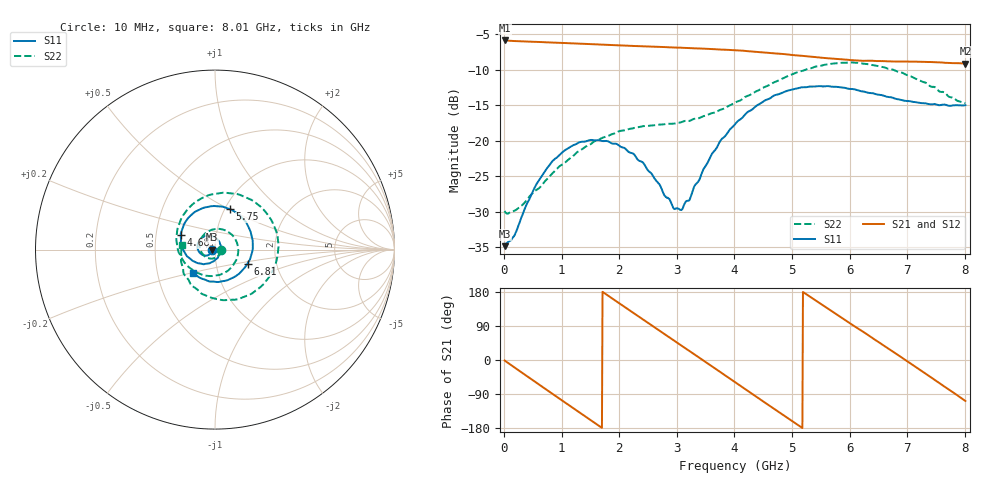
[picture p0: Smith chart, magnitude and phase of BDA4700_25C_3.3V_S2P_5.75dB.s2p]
!Agilent Technologies,E5071B,MY42404982,A.09.10
!Date: Mon Oct 20 18:05:24 2025
!Data & Calibration Information:
!Freq	S11:SOLT2(ON)	S21:SOLT2(ON)	S12:SOLT2(ON)	S22:SOLT2(ON)
# Hz S RI R 50
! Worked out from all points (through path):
!   801 points, 10 MHz to 8.01 GHz, reference 50 ohm
!   highest |S21| = -5.87 dB at 10 MHz (marker M1); lowest = -9.1 dB at 8.01 GHz (marker M2)
!   group delay of S21, straight-line fit = 286 ps
!   lowest |S11| = -34.8 dB at 10 MHz (marker M3), VSWR 1.04, Z = 48.2 - j0.106 ohm
!   |S11| at or under -10 dB: start of sweep to end of sweep
!   |S22| runs from -30.3 to -8.9 dB; largest |S21 - S12| = 0.0061
!   S11 on the Smith chart (normalised r, x): 10 MHz: 0.96, -0.00; 4.68 GHz: 0.67, +0.11; 5.75 GHz: 1.06, +0.51; 6.81 GHz: 1.42, -0.23; 8.01 GHz: 0.76, -0.20
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1e7  -0.0181 -0.0011  0.5086 -0.0111  0.5084 -0.0116  0.032 -0.00251
3.3e8  -0.0237 -0.02  0.4085 -0.2903  0.4083 -0.2903  0.023 -0.0273
7.1e8  -0.051 -0.0336  0.1238 -0.4786  0.1237 -0.4786  -0.0137 -0.0501
1.02e9  -0.0807 -0.0221  -0.1512 -0.4643  -0.1512 -0.4647  -0.0575 -0.0371
1.35e9  -0.0979 0.0111  -0.383 -0.2929  -0.383 -0.2934  -0.0853 0.0179
1.64e9  -0.0899 0.0467  -0.4732 -0.0599  -0.4733 -0.0597  -0.0673 0.0767
1.93e9  -0.0623 0.0724  -0.4339 0.1842  -0.4338 0.1845  -0.00695 0.1131
2.32e9  -0.0129 0.0727  -0.2082 0.4149  -0.208 0.415  0.0882 0.0881
2.68e9  0.0242 0.0441  0.0844 0.4508  0.0837 0.4506  0.1297 -0.00255
3.08e9  0.0304 -0.0118  0.3571 0.2776  0.3541 0.2797  0.0841 -0.1062
3.53e9  -0.0146 -0.0681  0.4391 -0.0656  0.4394 -0.0662  -0.0417 -0.1463
4.01e9  -0.111 -0.0694  0.2275 -0.3701  0.2281 -0.369  -0.1724 -0.0692
4.34e9  -0.1701 -0.0135  -0.0195 -0.4237  -0.0197 -0.4247  -0.2141 0.0439
4.68e9  -0.1913 0.0809  -0.2547 -0.3252  -0.254 -0.3266  -0.1848 0.1789
5.02e9  -0.1485 0.1769  -0.3838 -0.1169  -0.3851 -0.1174  -0.0717 0.2874
5.35e9  -0.0544 0.2349  -0.3734 0.1142  -0.374 0.1119  0.0912 0.3129
5.75e9  0.0848 0.2249  -0.2038 0.3182  -0.2032 0.3182  0.2775 0.2151
6.19e9  0.1897 0.1189  0.0711 0.3593  0.0758 0.3594  0.3509 -0.0138
6.68e9  0.1992 -0.0403  0.3161 0.1773  0.3171 0.1766  0.2232 -0.2317
6.81e9  0.1811 -0.0776  0.3472 0.1009  0.348 0.0983  0.165 -0.2618
7.5e9  0.00987 -0.1804  0.2058 -0.2922  0.2051 -0.2925  -0.137 -0.1918
8.01e9  -0.1231 -0.129  -0.109 -0.3326  -0.1083 -0.3332  -0.1823 0.0262
